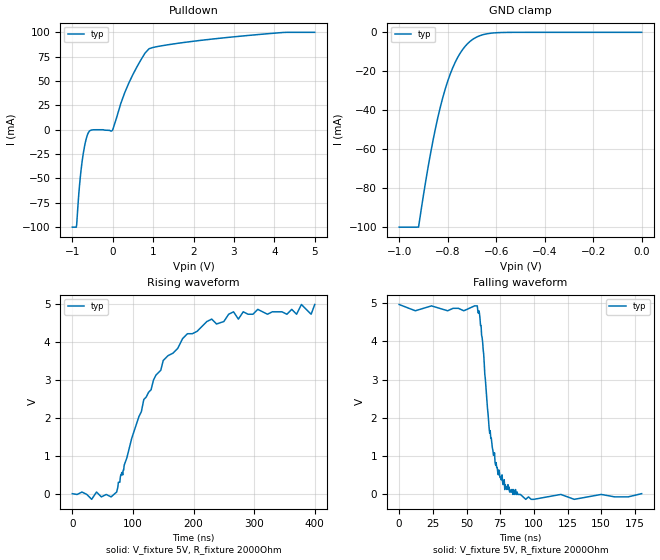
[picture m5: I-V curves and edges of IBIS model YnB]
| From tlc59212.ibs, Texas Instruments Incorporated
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|   Model YnB
[Model]   YnB
Model_type   Open_drain
Polarity   Inverting
Vmeas = 2.5
Vref = 5
Cref = 15pF
Rref = 2000
|   typ   min   max
C_comp   19p   NA   NA
[Voltage Range]   5   NA   NA
[Temperature Range]   27   NA   NA
[Pulldown Reference]   -0   NA   NA
[Power Clamp Reference]   5   NA   NA
[GND Clamp Reference]   -0   NA   NA
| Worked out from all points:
|   slope of the pulldown table from 0 to 0.75 V, typ, clamps not added: 9.94 ohm
|   GND clamp passes 1 mA (typ) near -0.65 V on its own axis
|   falling waveform, V_fixture 5V, R_fixture 2000Ohm: 20-80 % time 8.95ns typ, NA min, NA max; typ from 4.96 V to 0.02 V
|   rising waveform, V_fixture 5V, R_fixture 2000Ohm: 20-80 % time 88.1ns typ, NA min, NA max; typ from 0.02 V to 4.99 V
[Pulldown]
|   Voltage   I(typ)   I(min)   I(max)
-1V       -100mA     NA         NA
-900mV    -100mA     NA         NA
-830mV    -61.66mA   NA         NA
-780mV    -40.43mA   NA         NA
-700mV    -17.81mA   NA         NA
-620mV    -4.699mA   NA         NA
-520mV    -209.7uA   NA         NA
0V        -171.8uA   NA         NA
400mV     48mA       NA         NA
900mV     83.15mA    NA         NA
2.9V      94.97mA    NA         NA
5V        100mA      NA         NA
[GND Clamp]
|   Voltage   I(typ)   I(min)   I(max)
-1V       -100mA     NA         NA
-920mV    -99.97mA   NA         NA
-870mV    -61.83mA   NA         NA
-850mV    -49.17mA   NA         NA
-820mV    -33.48mA   NA         NA
-800mV    -25.18mA   NA         NA
-770mV    -15.68mA   NA         NA
-740mV    -9.141mA   NA         NA
-710mV    -4.907mA   NA         NA
-660mV    -1.423mA   NA         NA
-600mV    -221.7uA   NA         NA
0V        0A         NA         NA
[Ramp]
R_load = 2000
|   typ   min   max
dV/dt_r   2.9196/7.8e-08   NA   NA
dV/dt_f   2.994/8.6e-09   NA   NA
[Falling Waveform]
V_fixture = 5V
R_fixture = 2000Ohm
C_fixture = 0F
|   Time   V(typ)   V(min)   V(max)
0s        4.964V     NA         NA
58ns      4.928V     NA         NA
60.8ns    4.416V     NA         NA
67.2ns    1.6V       NA         NA
71.6ns    768mV      NA         NA
77.2ns    256mV      NA         NA
78ns      384mV      NA         NA
78.4ns    128mV      NA         NA
94ns      -128mV     NA         NA
180ns     20mV       NA         NA
[Rising Waveform]
V_fixture = 5V
R_fixture = 2000Ohm
C_fixture = 0F
|   Time   V(typ)   V(min)   V(max)
0s        20mV       NA         NA
73.2ns    64mV       NA         NA
118ns     2.496V     NA         NA
150ns     3.52V      NA         NA
190ns     4.224V     NA         NA
266ns     4.8V       NA         NA
370ns     4.736V     NA         NA
378ns     4.992V     NA         NA
394ns     4.736V     NA         NA
400ns     4.992V     NA         NA
